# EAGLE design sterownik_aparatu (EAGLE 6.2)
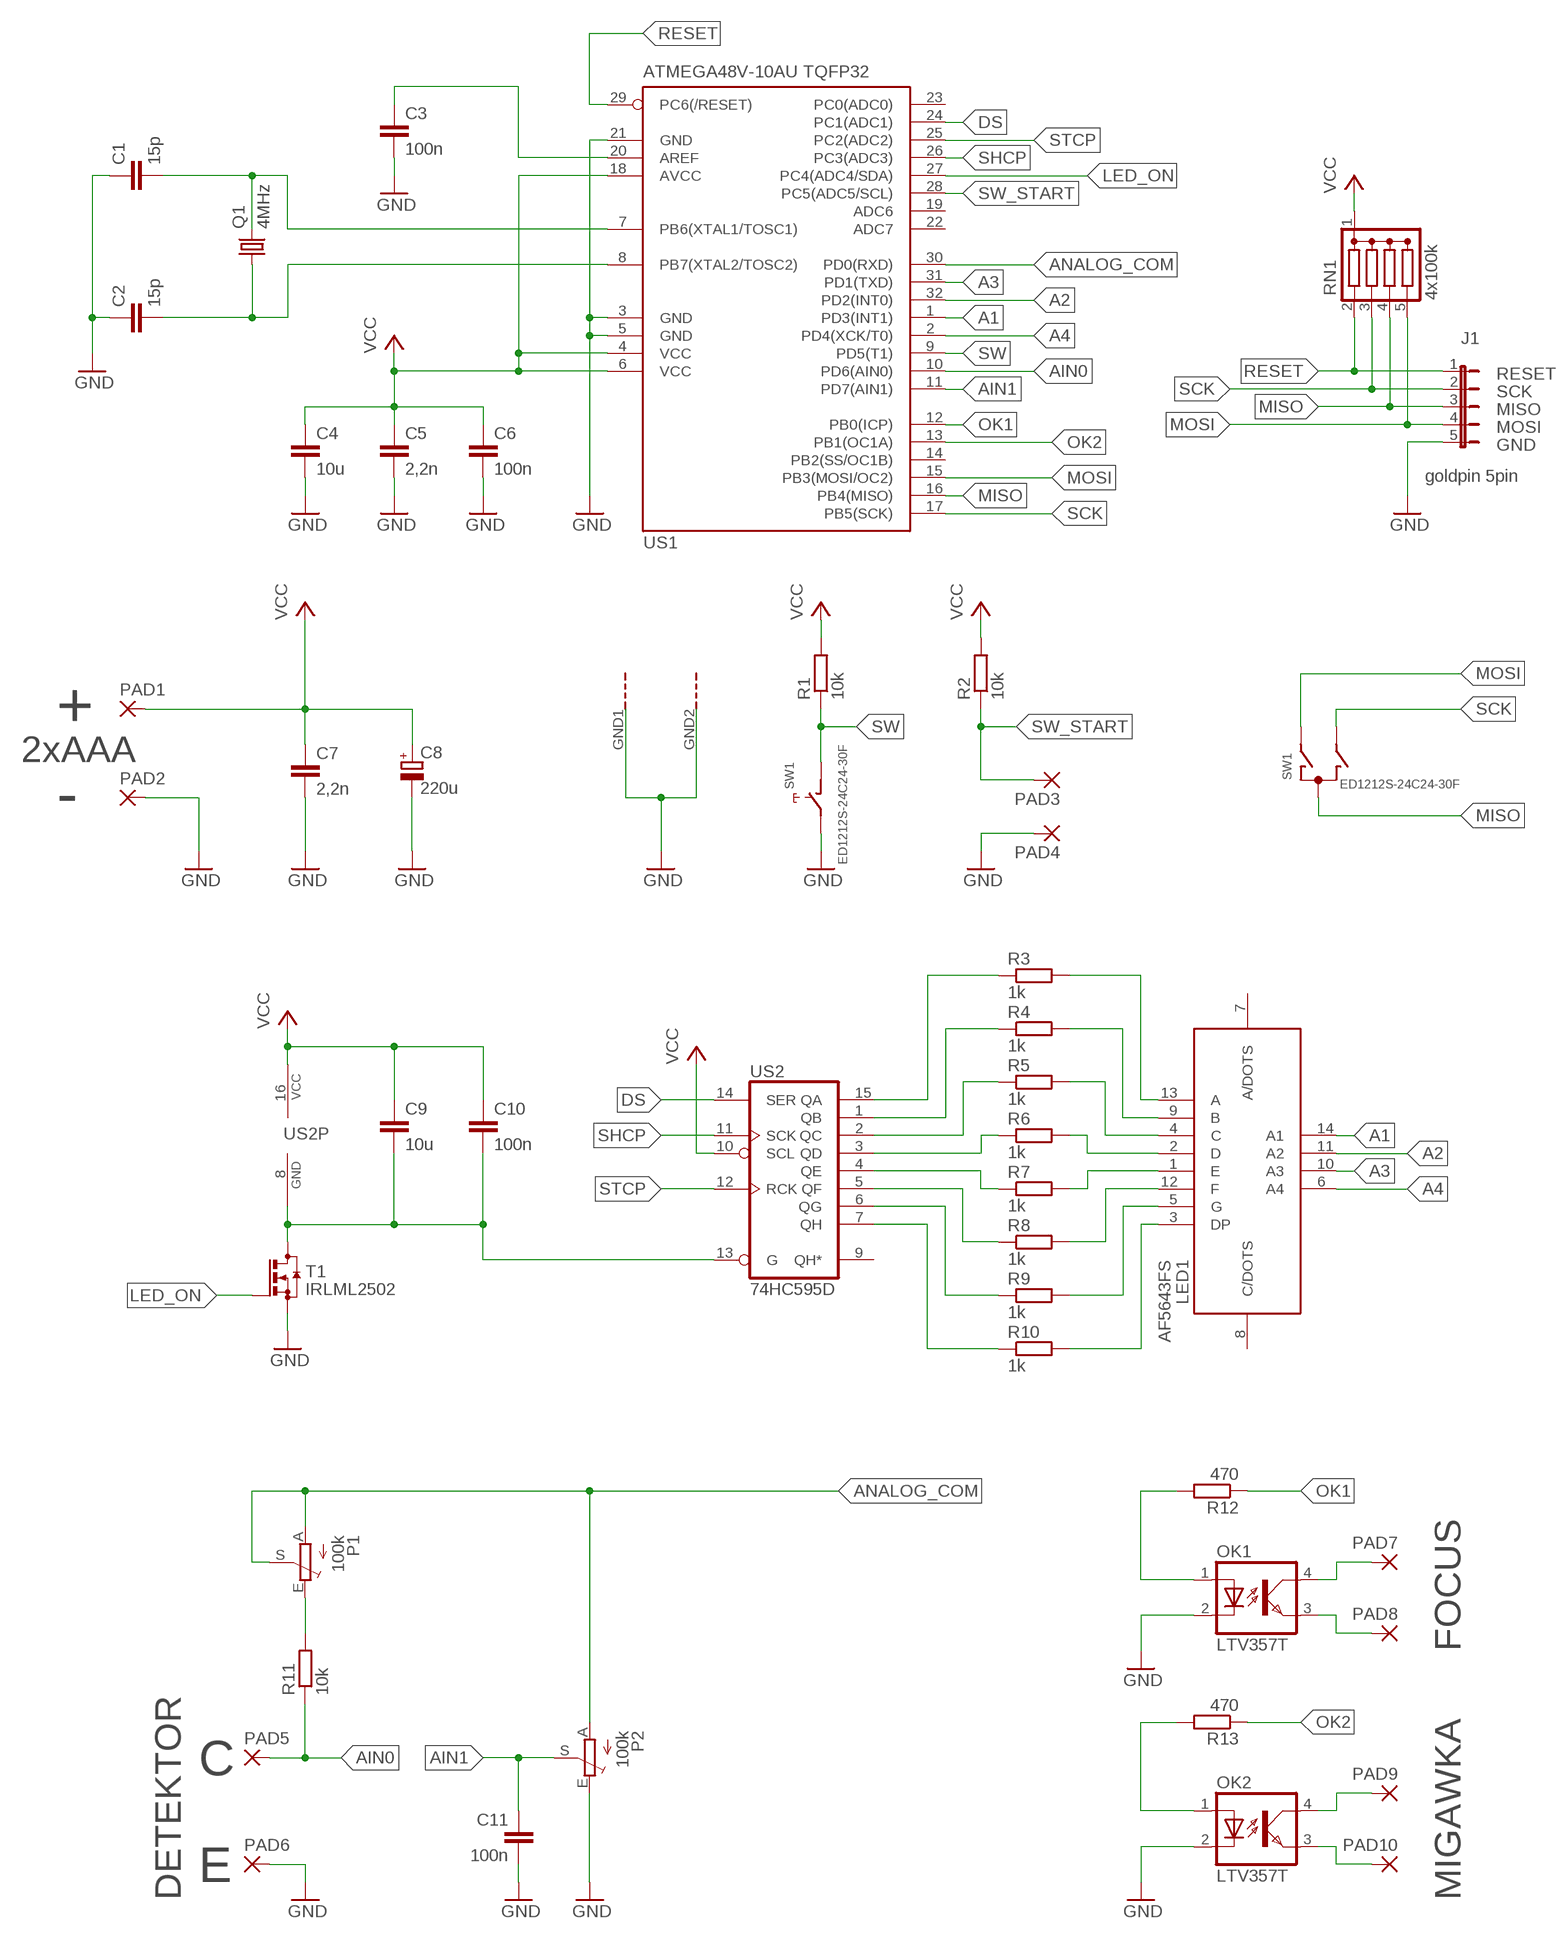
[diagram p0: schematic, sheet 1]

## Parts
C1  15p  C-EUC0805  [C0805]
C2  15p  C-EUC0805  [C0805]
C3  100n  C-EUC0805  [C0805]
C4  10u  C-EUC0805  [C0805]
C5  2,2n  C-EUC0805  [C0805]
C6  100n  C-EUC0805  [C0805]
C7  2,2n  C-EUC0805  [C0805]
C8  220u  CPOL-EUTT2D6L  [TT2D6L]
C9  10u  C-EUC0805  [C0805]
C10  100n  C-EUC0805  [C0805]
C11  100n  C-EUC0805  [C0805]
J1  goldpin 5pin  JUMPER-1X5  [JP5]
LED1  AF5643FS  LED_DISP_AF5643FS  [LED_DISP_AF5643FS]
OK1  LTV357T  LTV816S  [SMD4]
OK2  LTV357T  LTV816S  [SMD4]
P1  100k  TRIM_EU-CA6V  [CA6V]
P2  100k  TRIM_EU-CA6V  [CA6V]
PAD1  SMD5  [SMD2,54-5,08]
PAD2  SMD5  [SMD2,54-5,08]
PAD3  SMD5  [SMD2,54-5,08]
PAD4  SMD5  [SMD2,54-5,08]
PAD5  SMD5  [SMD2,54-5,08]
PAD6  SMD5  [SMD2,54-5,08]
PAD7  WIREPADSMD2,5X4MM  [SMD2,5X4MM]
PAD8  WIREPADSMD2,5X4MM  [SMD2,5X4MM]
PAD9  WIREPADSMD2,5X4MM  [SMD2,5X4MM]
PAD10  WIREPADSMD2,5X4MM  [SMD2,5X4MM]
Q1  4MHz  CRYSTALHC49U-V  [HC49U-V]
R1  10k  R-EU_R0805  [R0805]
R2  10k  R-EU_R0805  [R0805]
R3  1k  R-EU_R0805  [R0805]
R4  1k  R-EU_R0805  [R0805]
R5  1k  R-EU_R0805  [R0805]
R6  1k  R-EU_R0805  [R0805]
R7  1k  R-EU_R0805  [R0805]
R8  1k  R-EU_R0805  [R0805]
R9  1k  R-EU_R0805  [R0805]
R10  1k  R-EU_R0805  [R0805]
R11  10k  R-EU_R0805  [R0805]
R12  470  R-EU_R0805  [R0805]
R13  470  R-EU_R0805  [R0805]
RN1  4x100k  DRAB_REZ_1X4  [RN-5]
SW1  ED1212S-24C24-30F  EC12E_SW  [ALPS_EC12E_SW]
T1  IRLML2502  BSS123  [SOT23]
US1  ATMEGA48V-10AU TQFP32  MEGA8-AI  [TQFP32-08]
US2  74HC595D  74LS595D  [SO16]

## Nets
A1: LED1.14(A1) US1.1(PD3(INT1))
A2: LED1.11(A2) US1.32(PD2(INT0))
A3: LED1.10(A3) US1.31(PD1(TXD))
A4: LED1.6(A4) US1.2(PD4(XCK/T0))
AIN0: PAD5.1(P) R11.1 US1.10(PD6(AIN0))
AIN1: C11.1 P2.S US1.11(PD7(AIN1))
ANALOG_COM: P1.A P1.S P2.A US1.30(PD0(RXD))
DS: US1.24(PC1(ADC1)) US2.14(SER)
GND: C1.1 C2.1 C3.2 C4.2 C5.2 C6.2 C7.2 C8.- C11.2 J1.5 OK1.2(C) OK2.2(C) P2.E PAD2.1(P) PAD4.1(P) PAD6.1(P) SW1.E SW1.GND1(G) SW1.GND2(G) T1.2(S) US1.3(GND) US1.5(GND) US1.21(GND)
LED_ON: T1.1(G) US1.27(PC4(ADC4/SDA))
MISO: J1.3 RN1.4 SW1.C US1.16(PB4(MISO))
MOSI: J1.4 RN1.5 SW1.A US1.15(PB3(MOSI/OC2))
N$1: C2.2 Q1.1 US1.8(PB7(XTAL2/TOSC2))
N$2: C1.2 Q1.2 US1.7(PB6(XTAL1/TOSC1))
N$3: C3.1 US1.20(AREF)
N$4: C9.2 C10.2 T1.3(D) US2.8(GND) US2.13(G)
N$5: OK1.1(A) R12.2
N$6: P1.E R11.2
N$7: LED1.13(A) R3.2
N$8: LED1.9(B) R4.2
N$9: LED1.4(C) R5.2
N$10: LED1.2(D) R6.2
N$11: LED1.1(E) R7.2
N$12: LED1.12(F) R8.2
N$13: LED1.5(G) R9.2
N$14: LED1.3(DP) R10.2
N$15: OK1.4(COL) PAD7.P$1(P)
N$16: OK1.3(EMIT) PAD8.P$1(P)
N$17: OK2.1(A) R13.2
N$18: OK2.4(COL) PAD9.P$1(P)
N$19: OK2.3(EMIT) PAD10.P$1(P)
N$20: R6.1 US2.3(QD)
N$21: R7.1 US2.4(QE)
N$22: R8.1 US2.5(QF)
N$23: R5.1 US2.2(QC)
N$24: R9.1 US2.6(QG)
N$25: R4.1 US2.1(QB)
N$26: R3.1 US2.15(QA)
N$27: R10.1 US2.7(QH)
OK1: R12.1 US1.12(PB0(ICP))
OK2: R13.1 US1.13(PB1(OC1A))
RESET: J1.1 RN1.2 US1.29(PC6(/RESET))
SCK: J1.2 RN1.3 SW1.B US1.17(PB5(SCK))
SHCP: US1.26(PC3(ADC3)) US2.11(SCK)
STCP: US1.25(PC2(ADC2)) US2.12(RCK)
SW: R1.1 SW1.D US1.9(PD5(T1))
SW_START: PAD3.1(P) R2.1 US1.28(PC5(ADC5/SCL))
VCC: C4.1 C5.1 C6.1 C7.1 C8.+ C9.1 C10.1 PAD1.1(P) R1.2 R2.2 RN1.1(C) US1.4(VCC) US1.6(VCC) US1.18(AVCC) US2.10(SCL) US2.16(VCC)
Unconnected: LED1.7(A/DOTS) LED1.8(C/DOTS) US1.14(PB2(SS/OC1B)) US1.19(ADC6) US1.22(ADC7) US1.23(PC0(ADC0)) US2.9(QH*)

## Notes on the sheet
- RESET
- SCK
- MISO
- MOSI
- GND
- +
- 2xAAA
- -
- FOCUS
- C
- E
- DETEKTOR | MIGAWKA

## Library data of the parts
C1-C7 C9-C11 = rcl:C-EU: CAPACITOR, European symbol
C8 = rcl:CPOL-EU: POLARIZED CAPACITOR, European symbol
J1 = zlacza_futrzak:JUMPER-1X5
LED1 = inne_futrzak:LED_DISP_AF5643FS
OK1 OK2 = optocoupler:LTV816: OPTO COUPLER Source: LITEON, LTV816.pdf; OC_FARNELL: unknown; OC_NEWARK: unknown
P1 P2 = pot:TRIM_EU-: POTENTIOMETER
PAD1-PAD6 = wirepad:SMD5: SMD PAD
PAD7-PAD10 = zlacza_futrzak:WIREPAD
Q1 = crystal:CRYSTAL: CRYSTAL; OC_FARNELL: 1666969; OC_NEWARK: unknown
R1-R13 = rcl:R-EU_: RESISTOR, European symbol
RN1 = inne_futrzak:DRAB_REZ_1X4
SW1 = switch-alps:EC12E_SW: ALPS rotary Encoder EC12E series with switch; MPN: EC12E2424407; OC_FARNELL: 1520813; OC_NEWARK: 74M1068
T1 = transistor-small-signal:BSS123: N-CHANNEL MOS FET
US1 = atmel:MEGA8: MICROCONTROLLER 8 Kbytes FLASH, 1 kbytes SRAM, 512 bytes EEPROM, USART, 6-channel 10 bit ADC, 2-channel 8 bit ADC Pin compatible with Atmega48, ATMega88, ATMega168 Source: avr.lbr; MPN: ATMEGA8-16AU; OC_FARNELL: 9171371; OC_NEWARK: 73M8863
US2 = scalaki_futrzak:74*595: 8-bit SHIFT REGISTER, output latch

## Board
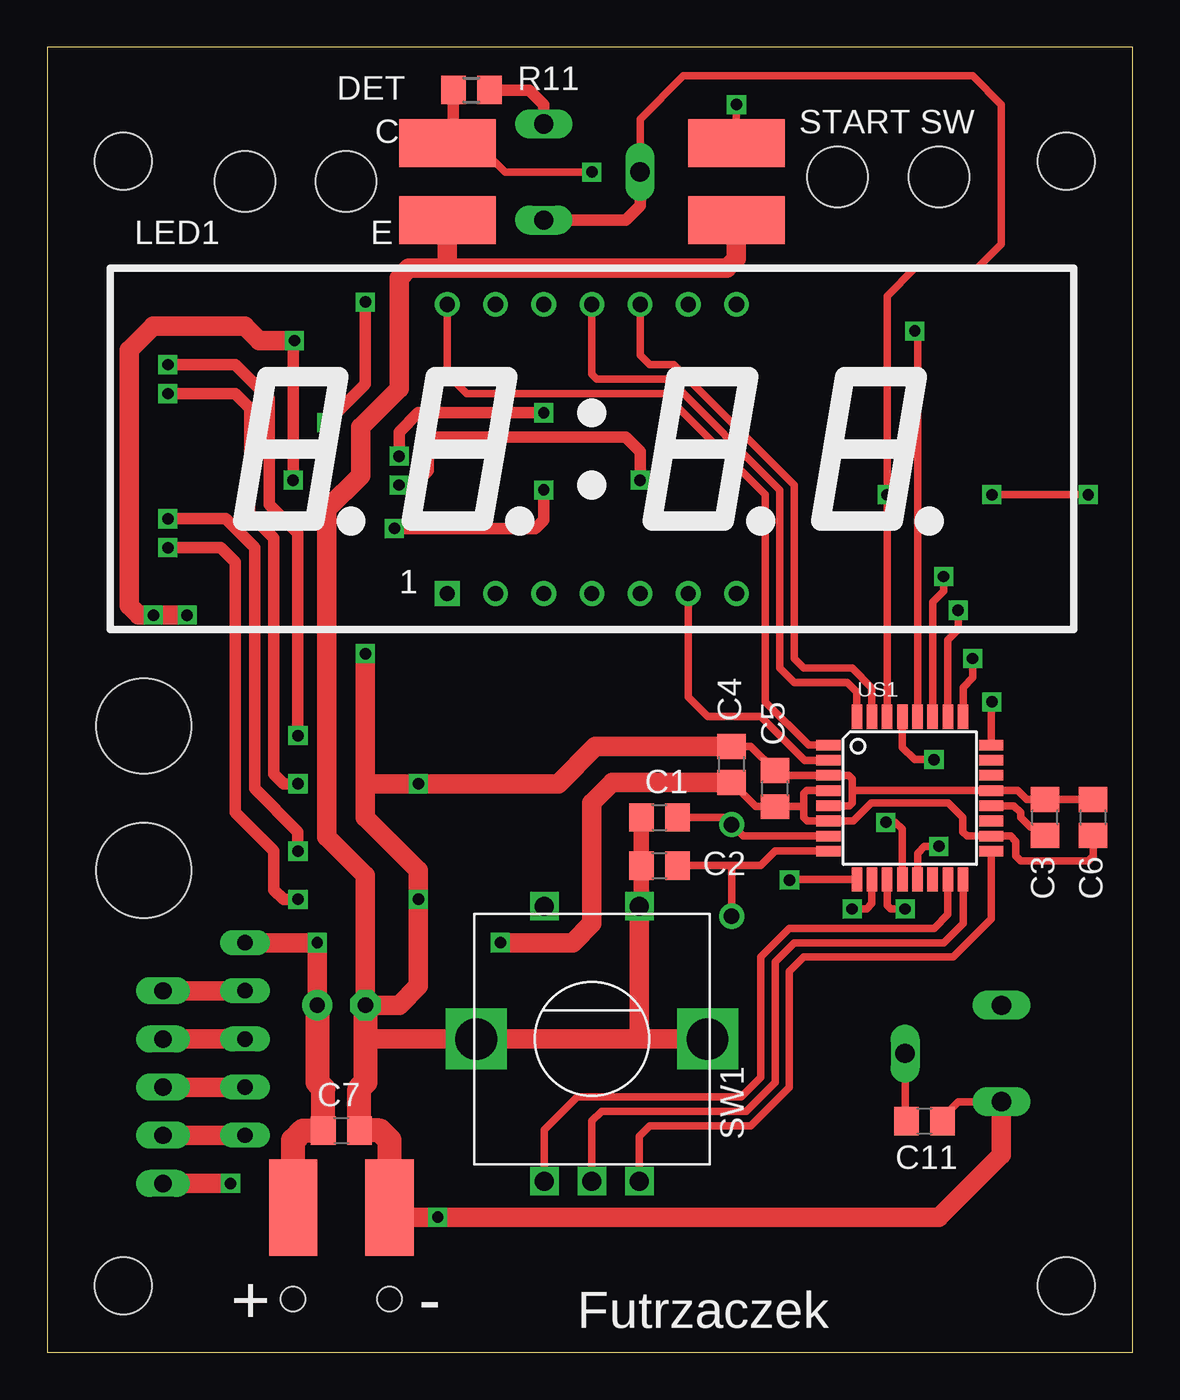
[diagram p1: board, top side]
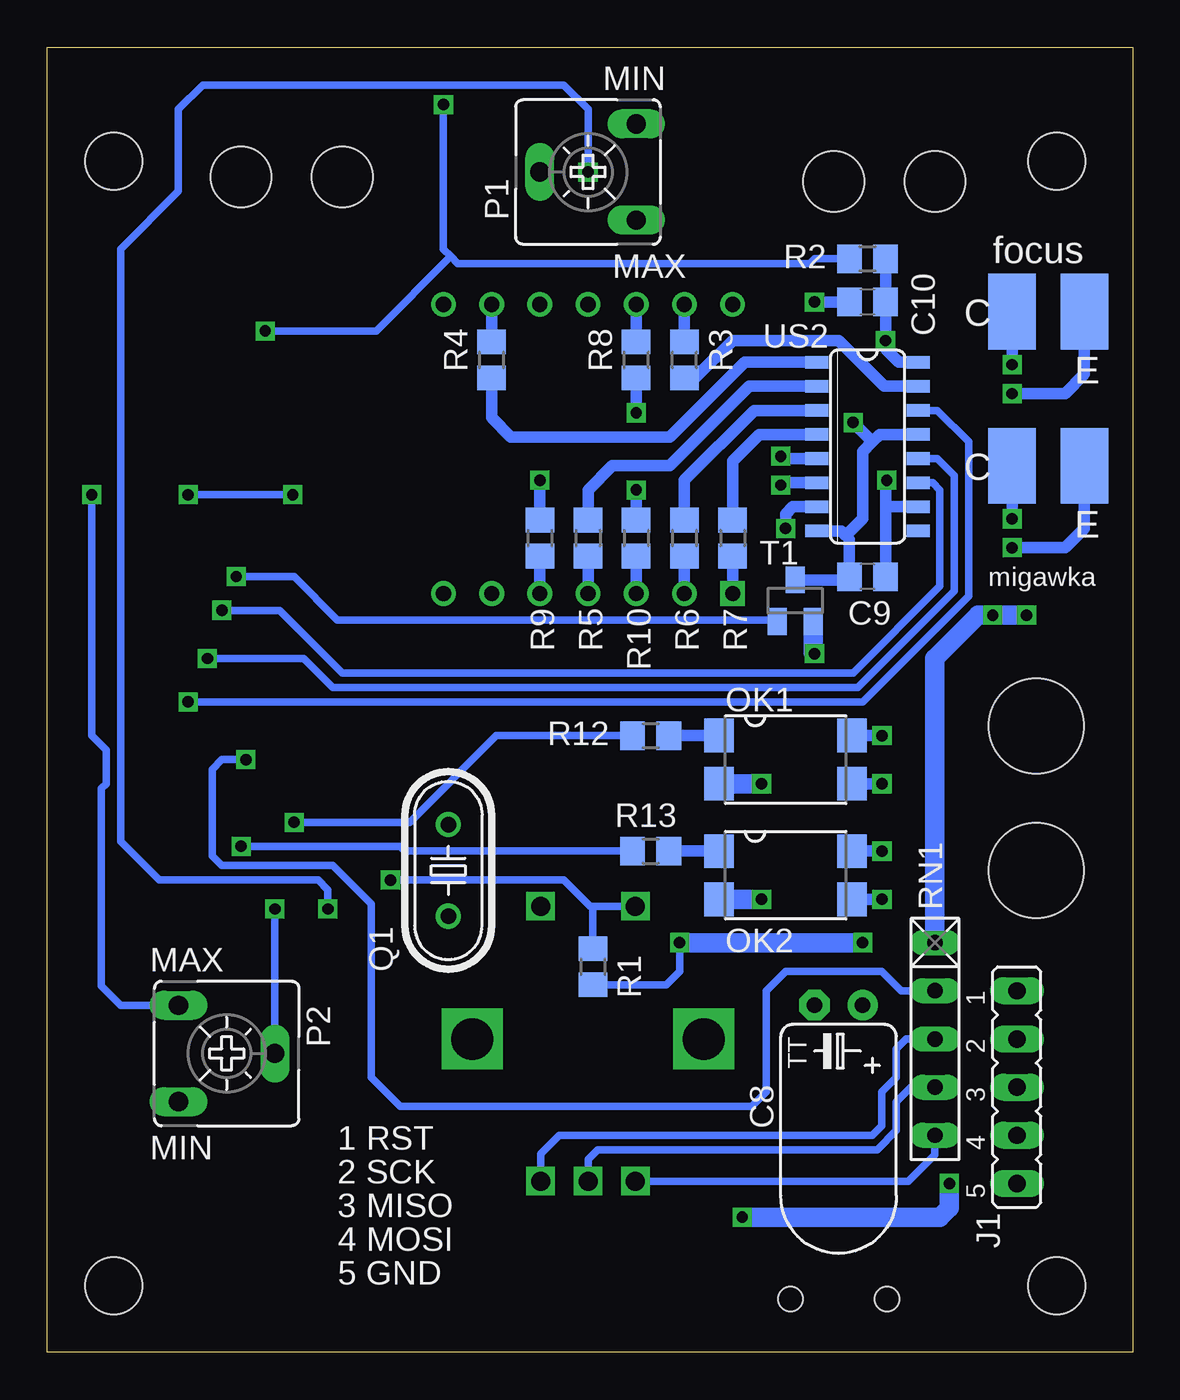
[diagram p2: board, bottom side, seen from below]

Size 57.2 x 68.8 mm. Coordinates in mm from the lower left corner, seen from the top.
Outline: 0,0 57.2,0 57.2,68.8 0,68.8 0,0
Copper layers (1*16): Top 0.035mm / dielectric 1.5mm / Bottom 0.035mm
Design rules: minimum track width 10mil, minimum drill 23mil, track to track 8mil, track to pad 8mil, pad to pad 8mil, via to via 8mil, smd to smd 8mil, copper to edge 40mil, drill to drill 8mil, minimum pad ring 10mil, minimum via ring 8mil, stop-mask expansion 4mil, vias tented up to drill 0mil, thermal gap 10mil
Holes 3 mm at 4,3.5 53.7,3.5 4,62.8 53.7,62.8
Holes 3.2 mm at 15.75,61.72 10.41,61.72 41.66,61.98 46.99,61.98
Holes 1.3 mm at 12.95,2.79 18.03,2.79
Holes 5 mm at 5.08,33.02 5.08,25.4

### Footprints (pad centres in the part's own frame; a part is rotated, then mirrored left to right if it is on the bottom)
C0805 = smd 1.3 x 1.5: 1 -0.95,0; 2 0.95,0
TT2D6L = drill 0.813 pad 1.6: + -1.27,0 | drill 0.813 pad 1.6 octagon: - 1.27,0
JP5 = drill 0.914 long: 1 -3.81,0; 2 -1.27,0; 3 1.27,0; 4 3.81,0; 5 6.35,0
LED_DISP_AF5643FS = drill 0.8 square: 1 17.78,1.905 | drill 0.8: 2 20.32,1.905; 3 22.86,1.905; 4 25.4,1.905; 5 27.94,1.905; 6 30.48,1.905; 7 33.02,1.905; 8 33.02,17.145; 9 30.48,17.145; 10 27.94,17.145; 11 25.4,17.145; 12 22.86,17.145; 13 20.32,17.145; 14 17.78,17.145
SMD4 = smd 1.78 x 1.55: 1 -1.27,-3.5; 2 1.27,-3.5; 3 1.27,3.5; 4 -1.27,3.5
CA6V = drill 1.016 long: A -2.54,-2.54; E 2.54,-2.54; S 0,2.54
SMD2,54-5,08 = smd 2.54 x 5.08: 1 0,0
SMD2,5X4MM = smd 2.5 x 4: P$1 0,0
HC49U-V = drill 0.813: 1 -2.413,0; 2 2.413,0
R0805 = smd 1.3 x 1.5: 1 -0.95,0; 2 0.95,0
RN-5 = drill 0.813 long: 1 -5.08,0; 2 -2.54,0; 3 0,0; 4 2.54,0; 5 5.08,0
ALPS_EC12E_SW = drill 1 square: A -2.5,-7.5; B 2.5,-7.5; C 0,-7.5; D -2.5,7; E 2.5,7 | drill 2.2 square: GND1 -6.1,0; GND2 6.1,0
SOT23 = smd 1 x 1.4: 1 -0.95,-1.1; 2 0.95,-1.1; 3 0,1.1
TQFP32-08 = smd 1.27 x 0.559: 1 -4.293,2.8; 2 -4.293,2; 3 -4.293,1.2; 4 -4.293,0.4; 5 -4.293,-0.4; 6 -4.293,-1.2; 7 -4.293,-2; 8 -4.293,-2.8; 17 4.293,-2.8; 18 4.293,-2; 19 4.293,-1.2; 20 4.293,-0.4; 21 4.293,0.4; 22 4.293,1.2; 23 4.293,2; 24 4.293,2.8 | smd 0.559 x 1.27: 9 -2.8,-4.293; 10 -2,-4.293; 11 -1.2,-4.293; 12 -0.4,-4.293; 13 0.4,-4.293; 14 1.2,-4.293; 15 2,-4.293; 16 2.8,-4.293; 25 2.8,4.293; 26 2,4.293; 27 1.2,4.293; 28 0.4,4.293; 29 -0.4,4.293; 30 -1.2,4.293; 31 -2,4.293; 32 -2.8,4.293
SO16 = smd 0.66 x 1.2: 1 -4.445,-2.673; 2 -3.175,-2.673; 3 -1.905,-2.673; 4 -0.635,-2.673; 5 0.635,-2.673; 6 1.905,-2.673; 7 3.175,-2.673; 8 4.445,-2.673; 9 4.445,2.673; 10 3.175,2.673; 11 1.905,2.673; 12 0.635,2.673; 13 -0.635,2.673; 14 -1.905,2.673; 15 -3.175,2.673; 16 -4.445,2.673

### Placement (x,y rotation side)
C1  32.26,28.19 0 top
C2  32.26,25.65 0 top
C3  52.58,28.19 90 top
C4  36.07,30.99 90 top
C5  38.35,29.72 90 top
C6  55.12,28.19 90 top
C7  15.49,11.68 0 top
C8  15.49,18.29 180 bottom
C9  13.97,40.89 180 bottom
C10  13.97,55.37 180 bottom
C11  46.23,12.19 0 top
J1  6.1,15.24 270 bottom
LED1  3.3,38.1 0 top
OK1  18.29,31.24 270 bottom
OK2  18.29,25.15 270 bottom
P1  28.7,62.23 90 bottom
P2  47.75,15.75 270 bottom
PAD1  12.95,7.62 0 top
PAD2  18.03,7.62 0 top
PAD3  36.32,63.75 90 top
PAD4  36.32,59.69 90 top
PAD5  21.08,63.75 90 top
PAD6  21.08,59.69 90 top
PAD7  6.35,54.86 180 bottom
PAD8  2.54,54.86 180 bottom
PAD9  6.35,46.74 0 bottom
PAD10  2.54,46.74 0 bottom
Q1  36.07,25.4 90 bottom
R1  28.45,20.32 270 bottom
R2  13.97,57.66 0 bottom
R3  23.62,52.32 90 bottom
R4  33.78,52.32 90 bottom
R5  28.7,42.93 270 bottom
R6  23.62,42.93 270 bottom
R7  21.08,42.93 270 bottom
R8  26.16,52.32 90 bottom
R9  31.24,42.93 270 bottom
R10  26.16,42.93 270 bottom
R11  22.35,66.55 0 top
R12  25.4,32.51 0 bottom
R13  25.4,26.42 0 bottom
RN1  10.41,16.51 270 bottom
SW1  28.7,16.51 0 top
T1  17.78,39.62 0 bottom
US1  45.47,29.21 0 top
US2  13.97,47.75 270 bottom

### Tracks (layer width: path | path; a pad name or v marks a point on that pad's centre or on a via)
A1
  Top 0.406: LED1.14 21.08,51.56 22.1,50.55 32.51,50.55 37.85,45.21 37.85,34.29 40.13,32.01 US1.1
A2
  Top 0.406: LED1.11 28.7,51.56 28.96,51.31 32.77,51.31 38.61,45.47 38.61,36.07 39.37,35.31 42.16,35.31 42.67,34.8 US1.32
A3
  Top 0.406: US1.31 43.47,35.02 42.42,36.07 39.88,36.07 39.37,36.58 39.37,45.72 33.02,52.07 31.75,52.07 31.24,52.58 LED1.10
A4
  Top 0.406: US1.2 39.91,31.21 37.59,33.53 34.8,33.53 33.78,34.54 LED1.6
AIN0  (via drill 0.6)
  Top 0.406: PAD5.1 22.61,63.75 24.13,62.23 v28.7,62.23 | US1.10 43.47,23.65 43.18,23.37 v42.42,23.37
  Top 0.61: R11.1 21.4,63.82 PAD5.1
  Bottom 0.406: v28.7,62.23 28.7,65.53 29.97,66.8 49.02,66.8 50.29,65.53 50.29,61.21 53.34,58.17 53.34,26.92 51.31,24.89 42.93,24.89 42.42,24.38 v42.42,23.37
AIN1  (via drill 0.6)
  Top 0.406: US1.11 44.27,23.55 44.45,23.37 v45.21,23.37 | P2.S 45.21,12.26 C11.1
  Bottom 0.406: v45.21,23.37 P2.S
ANALOG_COM  (via drill 0.6)
  Top 0.406: P1.S 31.24,65.02 33.53,67.31 48.77,67.31 50.29,65.79 50.29,58.42 49.02,57.15 45.72,57.15 44.27,55.7 v44.27,45.21 US1.30 | v54.86,45.21 v49.78,45.21
  Top 0.61: P1.A 30.48,59.69 31.24,60.45 P1.S
  Bottom 0.406: P2.A 53.34,18.29 54.36,19.3 54.36,29.72 54.1,29.97 54.1,31.75 54.86,32.51 v54.86,45.21 | v49.78,45.21 v44.27,45.21
DS  (via drill 0.6)
  Top 0.406: US1.24 49.76,34.27 v49.78,34.29
  Bottom 0.406: v49.78,34.29 14.22,34.29 8.64,39.88 8.64,48.01 10.29,49.66 US2.14
GND  (via drill 0.6)
  Top 0.406: 42.42,29.72 42.42,30.23 42.23,30.41 US1.3 38.61,30.41 C5.2 37.08,31.94 C4.2 | 42.42,29.72 42.42,28.96 42.27,28.81 US1.5 | 42.42,29.72 42.53,29.61 US1.21 51.16,29.61 51.63,29.14 C3.2 C6.2 | C11.2 47.18,12.38 48.01,13.21 P2.E
  Top 0.813: C1.1 C2.1 31.31,23.62 SW1.E
  Top 1.016: 21.08,57.15 19.05,57.15 18.54,56.64 18.54,50.8 16.51,48.77 16.51,46.23 14.73,44.45 14.73,27.18 16.76,25.15 C8.- 18.54,18.29 19.56,19.3 v19.56,23.88 19.56,25.4 16.76,28.19 16.76,29.97 | 21.08,57.15 35.81,57.15 36.32,57.66 PAD4.1 | PAD6.1 21.08,57.15 | SW1.GND2 31.5,16.51 | 31.5,16.51 SW1.GND1 | SW1.GND1 17.02,16.51 16.76,16.26 | SW1.E 31.2,16.8 31.5,16.51 | v16.76,36.83 16.76,29.97 | SW1.GND1 | J1.5 v9.65,8.89 | PAD2.1 18.54,7.11 v20.57,7.11 46.99,7.11 50.29,10.41 P2.E | 16.76,29.97 v19.56,29.97 26.92,29.97 28.89,31.94 C4.2
  Top 1.27: PAD2.1 18.03,11.18 17.53,11.68 C7.2 16.44,13.9 16.76,14.22 16.76,16.26 C8.-
  Bottom 1.016: v16.76,36.83 16.83,36.9 T1.2 | v9.65,8.89 9.65,7.62 10.16,7.11 v20.57,7.11 | OK2.2 v19.56,23.88 | OK1.2 v19.56,29.97
LED_ON  (via drill 0.6)
  Top 0.406: US1.27 46.67,39.55 47.24,40.13 v47.24,40.89
  Bottom 0.406: v47.24,40.89 44.2,40.89 41.91,38.61 18.81,38.61 T1.1
MISO
  Top 0.406: US1.16 48.27,22.61 47.24,21.59 39.37,21.59 38.35,20.57 38.35,14.22 36.83,12.7 29.21,12.7 28.7,12.19 SW1.C
  Top 1.016: J1.3 RN1.4
  Bottom 0.406: SW1.C 28.7,10.16 28.19,10.67 13.46,10.67 12.45,11.68 12.45,13.21 11.68,13.97 RN1.4
MOSI
  Top 0.406: US1.15 47.47,23.08 46.74,22.35 39.12,22.35 37.59,20.83 37.59,14.48 36.58,13.46 27.94,13.46 26.2,11.72 SW1.A
  Top 1.016: J1.4 RN1.5
  Bottom 0.406: RN1.5 10.41,10.41 11.82,9.01 SW1.A
N$1
  Top 0.406: C2.2 36.07,25.65 | 36.07,25.65 37.59,25.65 38.35,26.42 US1.8 | Q1.1 36.07,25.65
N$2
  Top 0.406: US1.7 36.67,27.21 Q1.2 35.69,28.19 C1.2
N$3
  Top 0.406: US1.20 50.95,28.81 51.31,28.45 51.31,28.19 51.82,27.69 52.14,27.69 C3.1
N$4  (via drill 0.6)
  Top 0.61: v16.76,55.37 16.76,51.05 v14.73,49.02
  Bottom 0.61: US2.8 15.37,43.31 15.11,43.05 | 15.11,43.05 14.92,42.86 C9.2 15.09,40.72 T1.3 | US2.13 13.34,48.39 13.72,48.01 | 13.72,48.01 14.22,47.5 14.22,43.94 15.11,43.05 | C10.2 v16.76,55.37 | v14.73,49.02 13.72,48.01
N$5
  Bottom 0.61: OK1.1 R12.2
N$6
  Top 0.61: R11.2 25.4,66.55 26.16,65.79 P1.E
N$7
  Bottom 0.61: R3.2 LED1.13
N$8
  Bottom 0.61: R4.2 LED1.9
N$9
  Bottom 0.61: R5.2 LED1.4
N$10
  Bottom 0.61: R6.2 LED1.2
N$11
  Bottom 0.61: R7.2 LED1.1
N$12
  Bottom 0.61: R8.2 LED1.12
N$13
  Bottom 0.61: R9.2 LED1.5
N$14
  Bottom 0.61: R10.2 LED1.3
N$15  (via drill 0.6)
  Top 0.61: v13.21,32.51 13.21,43.18 11.68,44.7 11.68,50.29 9.91,52.07 v6.35,52.07
  Bottom 0.61: OK1.4 v13.21,32.51 | PAD7.P$1 v6.35,52.07
N$16  (via drill 0.6)
  Top 0.61: v13.21,29.97 12.45,29.97 11.94,30.48 11.94,42.93 10.67,44.2 10.67,49.78 9.91,50.55 v6.35,50.55
  Bottom 0.61: OK1.3 v13.21,29.97 | PAD8.P$1 2.54,51.56 3.56,50.55 v6.35,50.55
N$17
  Bottom 0.61: OK2.1 R13.2
N$18  (via drill 0.6)
  Top 0.61: v6.35,43.94 9.4,43.94 10.92,42.42 10.92,29.72 13.21,27.43 v13.21,26.42
  Bottom 0.61: OK2.4 v13.21,26.42 | PAD9.P$1 v6.35,43.94
N$19  (via drill 0.6)
  Top 0.61: v6.35,42.42 9.14,42.42 9.91,41.66 9.91,28.45 11.94,26.42 11.94,24.38 12.45,23.88 v13.21,23.88
  Bottom 0.61: OK2.3 v13.21,23.88 | PAD10.P$1 2.54,43.43 3.56,42.42 v6.35,42.42
N$20
  Bottom 0.61: US2.3 19.94,49.66 23.62,45.97 R6.1
N$21
  Bottom 0.61: US2.4 19.68,48.39 21.08,46.99 R7.1
N$22  (via drill 0.6)
  Top 0.61: v26.16,49.53 19.56,49.53 18.54,48.51 v18.54,47.24
  Bottom 0.61: US2.5 18.41,47.12 v18.54,47.24 | v26.16,49.53 R8.1
N$23
  Bottom 0.61: US2.2 20.19,50.93 24.38,46.74 27.43,46.74 28.7,45.47 R5.1
N$24  (via drill 0.6)
  Top 0.61: v18.54,45.72 19.3,45.72 20.07,46.48 20.07,47.75 20.57,48.26 30.48,48.26 31.24,47.5 v31.24,45.97
  Bottom 0.61: US2.6 18.41,45.85 v18.54,45.72 | v31.24,45.97 R9.1
N$25
  Bottom 0.61: R4.1 33.78,49.28 32.77,48.26 24.38,48.26 20.45,52.2 US2.1
N$26
  Bottom 0.61: R3.1 23.05,51.37 21.08,53.34 15.49,53.34 13.08,50.93 US2.15
N$27  (via drill 0.6)
  Top 0.61: v18.29,43.43 25.72,43.43 R10.1 v26.16,45.47
  Bottom 0.61: US2.7 17.91,44.58 18.29,44.2 v18.29,43.43 | v26.16,45.47 R10.1
OK1  (via drill 0.6)
  Top 0.406: US1.12 45.07,27.58 44.7,27.94 v44.2,27.94
  Bottom 0.406: v44.2,27.94 38.1,27.94 33.53,32.51 R12.1
OK2  (via drill 0.6)
  Top 0.406: US1.13 45.87,26.31 46.23,26.67 v46.99,26.67
  Bottom 0.406: v46.99,26.67 38.61,26.67 38.35,26.42 R13.1
RESET  (via drill 0.6)
  Top 0.406: v46.74,31.24 45.72,31.24 45.07,31.9 US1.29
  Top 1.016: J1.1 RN1.2
  Bottom 0.406: RN1.2 12.19,19.05 13.21,20.07 18.29,20.07 19.3,19.05 19.3,13.72 20.07,12.95 38.61,12.95 40.13,14.48 40.13,23.62 42.16,25.65 48.01,25.65 48.51,26.16 48.51,30.73 48.01,31.24 v46.74,31.24
SCK
  Top 0.406: US1.17 49.76,22.84 47.75,20.83 39.88,20.83 39.12,20.07 39.12,13.97 37.08,11.94 31.75,11.94 31.2,11.39 SW1.B
  Top 1.016: RN1.3 J1.2
  Bottom 0.406: RN1.3 11.94,16.51 12.45,16 12.45,14.48 13.21,13.72 13.21,11.94 13.72,11.43 30.23,11.43 31.2,10.45 SW1.B
SHCP  (via drill 0.6)
  Top 0.406: US1.26 47.47,37.56 48.01,38.1 v48.01,39.12
  Bottom 0.406: v48.01,39.12 44.96,39.12 41.66,35.81 14.73,35.81 10.16,40.39 10.16,45.47 10.54,45.85 US2.11
STCP  (via drill 0.6)
  Top 0.406: US1.25 48.27,35.06 48.77,35.56 v48.77,36.58
  Bottom 0.406: v48.77,36.58 43.69,36.58 42.16,35.05 14.48,35.05 9.4,40.13 9.4,46.23 10.29,47.12 US2.12
SW  (via drill 0.6)
  Top 0.406: US1.9 39.14,24.92 v39.12,24.89
  Bottom 0.406: v39.12,24.89 29.97,24.89 28.59,23.51 | SW1.D 28.59,23.51 | R1.1 28.45,23.4 28.59,23.51
SW_START  (via drill 0.6)
  Top 0.406: v36.32,65.79 PAD3.1 | US1.28 45.87,53.7 v45.72,53.85
  Bottom 0.406: 35.94,57.78 35.56,57.4 17.02,57.4 16.76,57.66 R2.1 | 35.94,57.78 36.32,58.17 v36.32,65.79 | v45.72,53.85 39.88,53.85 35.94,57.78
VCC  (via drill 0.6)
  Top 0.406: 39.88,28.7 39.88,28.19 40.06,28.01 US1.6 42.49,28.01 43.43,28.96 47.5,28.96 48.26,28.19 48.26,27.43 48.48,27.21 US1.18 50.77,27.21 51.05,26.92 51.05,26.16 51.31,25.91 54.86,25.91 55.12,26.16 C6.1 | 39.88,28.7 39.88,29.46 40.02,29.61 US1.4 | 39.88,28.7 39.81,28.77 C5.1 37.34,28.77 C4.1
  Top 0.61: v12.95,45.97 12.95,53.27 v13.02,53.34
  Top 1.016: C8.+ v14.22,21.59 RN1.1 | v23.88,21.59 27.69,21.59 28.7,22.61 28.7,28.96 29.78,30.04 C4.1 | v13.02,53.34 11.18,53.34 10.41,54.1 5.59,54.1 4.32,52.83 4.32,39.37 4.83,38.86 v5.59,38.86 v7.37,38.86
  Top 1.27: PAD1.1 12.95,11.18 13.46,11.68 C7.1 14.54,13.9 14.22,14.22 C8.+
  Bottom 0.406: R1.2 24.57,19.37 23.88,20.07 v23.88,21.59
  Bottom 0.61: US2.10 12.89,44.58 13.02,44.7 | C9.1 13.02,44.7 | 13.02,44.7 13.02,45.91 v12.95,45.97 | US2.16 12.32,52.2 13.02,52.9 v13.02,53.34 C10.1 R2.2
  Bottom 1.016: v14.22,21.59 v23.88,21.59 | RN1.1 10.41,36.58 8.13,38.86 v5.59,38.86

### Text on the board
tPlace: DET | C | START SW | E | + | - | Futrzaczek
bPlace: MIN | focus | MAX | C | E | C | E | migawka | MAX | 1 RST | MIN | 2 SCK | 3 MISO | 4 MOSI | 5 GND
